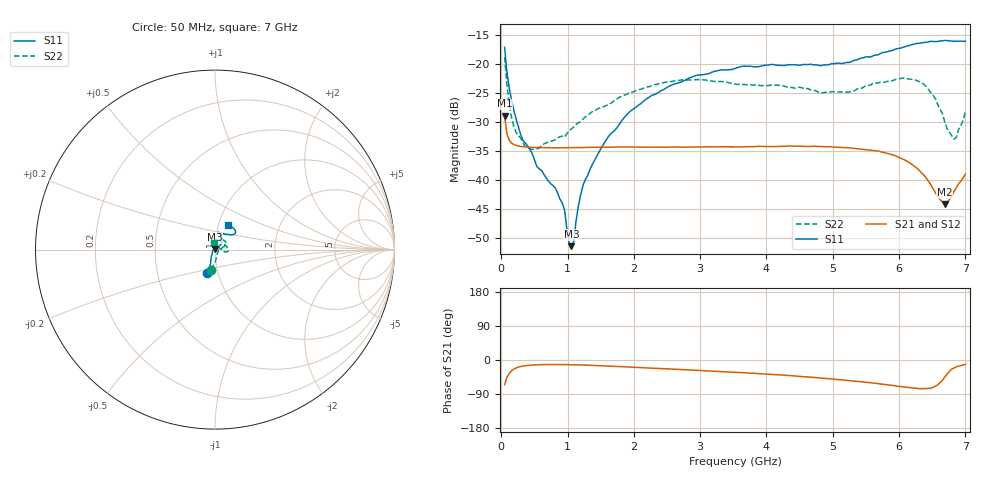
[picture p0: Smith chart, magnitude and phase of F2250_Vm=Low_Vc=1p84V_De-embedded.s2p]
! Integrated Device Technology
! Corporate Headquarters
! 6024 Silver Creek Valley Road
! San Jose, CA 95138  USA
! Phone:  1-408-284-8200
! Toll Free:  1-800-223-1366
! Webpage:  http://www.idt.com/
! Timing and RF Division
! 515 Groton Road, Suite 102
! Westford, MA 01886-6024
! Device:  F2250
! Description: Voltage Variable RF Attenuator
! Frequency:  50.0 -  6000.00 MHz
! Package:  3x3 mm Thin QFN Plastic Package: 16 pin
! Ports:  2 RF, 3 DC
!  Pin  1  = GND
!  Pin  2  = NC
!  Pin  3  = RF1  = Port 1
!  Pin  4  = NC
!  Pin  5  = GND
!  Pin  6  = GND
!  Pin  7  = GND
!  Pin  8  = GND
!  Pin  9  = NC
!  Pin 10  = RF2  = Port 2
!  Pin 11  = NC
!  Pin 12  = GND
!  Pin 13  = GND
!  Pin 14  = VCNTRL
!  Pin 15  = VDD
!  Pin 16  = VMODE
! Vcntrl:  1.840 Volts
! Vmode:  +0.000 Volts
! Vdd:  +3.30  Volts
! Current:  1.185 mA
! Data:  The device was measured on a the F2250 evaluation board which has
!  individual transmission lines to the RF pins.  Data was collected
!  using a calibrated network analyzer.  The evaluation board was
!  de-embedded using a TRL calibration technique.
!  The reference plane is the edge of the package pin.
! Misc:  SN 10
!  Action Tracker AT0258
! Date Measured:  2014-11-26
! Date:  2015-10-15  MJV
! Note:
!  Integrated Device Technology supplies this data as a sample of measured
!  data at the package pin for this product.  Your particular data for this
!  product may vary.
!  Data was taken at 25 degrees C.
!  Integrated Device Technology reserves the right to change this data at anytime.
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# GHz S dB R 50
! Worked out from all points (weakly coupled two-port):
!   201 points, 50 MHz to 7 GHz, reference 50 ohm
!   highest |S21| = -28.93 dB at 50 MHz (marker M1); lowest = -44.2 dB at 6.687 GHz (marker M2)
!   lowest |S11| = -51.4 dB at 1.058 GHz (marker M3), VSWR 1.01, Z = 49.9 + j0.235 ohm
!   |S11| at or under -10 dB: start of sweep to end of sweep
!   |S22| runs from -34.8 to -18.8 dB; largest |S21 - S12| = 5.3e-05
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0.05  -17.17 -108.4  -28.93 -65.0  -28.93 -65.0  -18.85 -101.9
0.08475  -21.44 -107.2  -32.07 -46.2  -32.06 -46.2  -23.62 -87.6
0.15425  -26.24 -116.2  -33.66 -28.5  -33.66 -28.5  -29.25 -74.5
0.29325  -32.23 -127.0  -34.25 -17.2  -34.24 -17.2  -32.82 -45.1
0.36275  -33.66 -138.4  -34.34 -15.0  -34.34 -15.0  -34.26 -29.5
0.91875  -43.97 158.1  -34.49 -12.1  -34.49 -12.1  -32.47 3.1
0.9535  -45.13 170.2  -34.49 -12.1  -34.49 -12.1  -32.64 5.7
1.023  -50.84 143.0  -34.48 -12.3  -34.48 -12.3  -31.54 8.3
1.05775  -51.42 118.5  -34.48 -12.4  -34.47 -12.4  -31.23 9.4
1.0925  -50.61 84.0  -34.46 -12.5  -34.47 -12.5  -30.90 9.1
1.162  -44.55 53.8  -34.45 -12.8  -34.45 -12.8  -30.19 8.2
1.2315  -40.98 42.3  -34.44 -13.1  -34.43 -13.2  -29.55 7.8
1.6485  -32.09 41.3  -34.38 -16.1  -34.38 -16.1  -26.85 17.0
2.37825  -24.88 47.1  -34.36 -22.3  -34.36 -22.4  -23.45 27.1
3.525  -20.82 72.3  -34.34 -32.5  -34.34 -32.5  -23.52 55.0
4.7065  -20.19 72.3  -34.22 -46.0  -34.22 -46.0  -24.60 59.6
5.22775  -19.80 56.3  -34.47 -54.0  -34.47 -54.1  -24.90 36.0
5.85325  -17.83 40.4  -35.54 -66.1  -35.54 -66.2  -22.96 3.8
6.3745  -16.34 41.3  -39.17 -75.6  -39.19 -75.7  -23.56 -10.8
6.68725  -16.00 48.7  -44.20 -45.3  -44.21 -45.0  -29.94 7.3
6.82625  -16.15 53.5  -42.04 -21.3  -42.02 -21.0  -32.99 50.0
7  -16.14 63.2  -39.00 -11.9  -38.97 -12.1  -28.23 99.6
